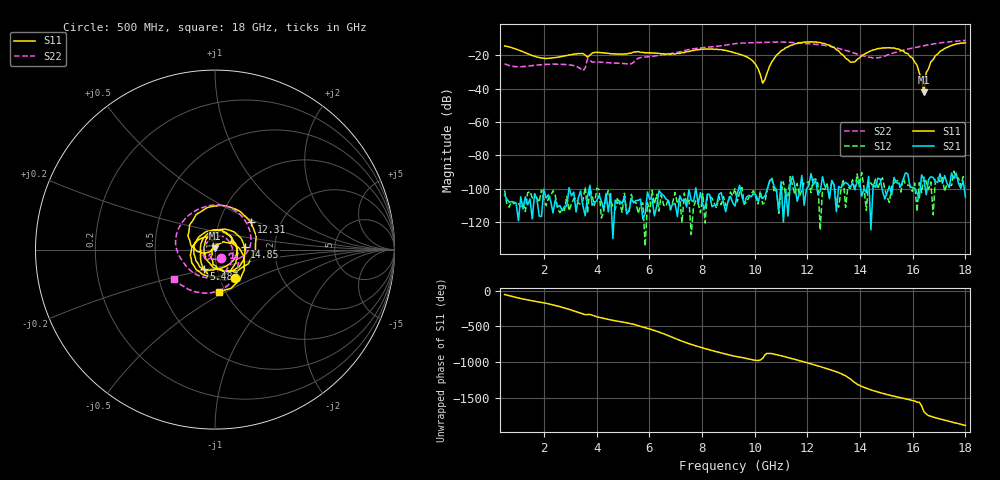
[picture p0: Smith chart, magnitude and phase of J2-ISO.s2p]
!Agilent Technologies,N5230C,MY49001096,A.09.42.15
!Agilent N5230C: A.09.42.15
!Date: Thursday, June 29, 2023 08:11:15
!Correction: S11(Full 2 Port(1,2))
!S21(Full 2 Port(1,2))
!S12(Full 2 Port(1,2))
!S22(Full 2 Port(1,2))
!S2P File: Measurements: S11, S21, S12, S22:
# Hz S  dB  R 50
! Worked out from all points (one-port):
!   201 points, 500 MHz to 18 GHz, reference 50 ohm
!   lowest |S11| = -42.2 dB at 16.43 GHz (marker M1), VSWR 1.02, Z = 49.8 + j0.735 ohm
!   |S11| at or under -10 dB: start of sweep to end of sweep
!   S11 on the Smith chart (normalised r, x): 500 MHz: 1.18, -0.38; 5.487 GHz: 0.86, -0.19; 12.31 GHz: 1.41, +0.46; 14.85 GHz: 1.40, +0.04; 18 GHz: 0.93, -0.47
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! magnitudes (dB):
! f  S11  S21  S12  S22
! 500 MHz  -14.4  -103.8  -101.0  -25.1
! 1.9 GHz  -21.7  -116.6  -100.7  -25.7
! 3.475 GHz  -18.9  -110.3  -106.9  -29.3
! 3.65 GHz  -21.1  -104.4  -113.8  -22.0
! 5.487 GHz  -18.0  -107.0  -108.1  -22.8
! 6.362 GHz  -18.8  -101.1  -113.3  -20.0
! 9.25 GHz  -18.5  -110.3  -99.8  -13.0
! 9.95 GHz  -23.8  -102.9  -101.1  -12.4
! 10.3 GHz  -36.7  -105.7  -109.2  -12.3
! 10.65 GHz  -23.9  -94.0  -93.2  -12.1
! 11 GHz  -17.3  -95.7  -102.3  -12.0
! 12.22 GHz  -12.0  -97.7  -94.4  -13.3
! 12.31 GHz  -12.0  -94.8  -94.0  -13.4
! 13.62 GHz  -24.1  -99.2  -99.8  -17.8
! 14.85 GHz  -15.6  -101.1  -93.3  -20.8
! 15.11 GHz  -15.4  -98.4  -108.1  -19.4
! 15.99 GHz  -21.6  -99.1  -101.5  -15.6
! 16.16 GHz  -25.9  -102.6  -113.6  -15.0
! 16.43 GHz  -42.2  -94.2  -93.0  -14.2
! 16.51 GHz  -30.3  -103.5  -95.7  -13.9
! 16.86 GHz  -20.1  -95.8  -94.3  -12.9
! 18 GHz  -12.4  -104.9  -93.4  -11.1
